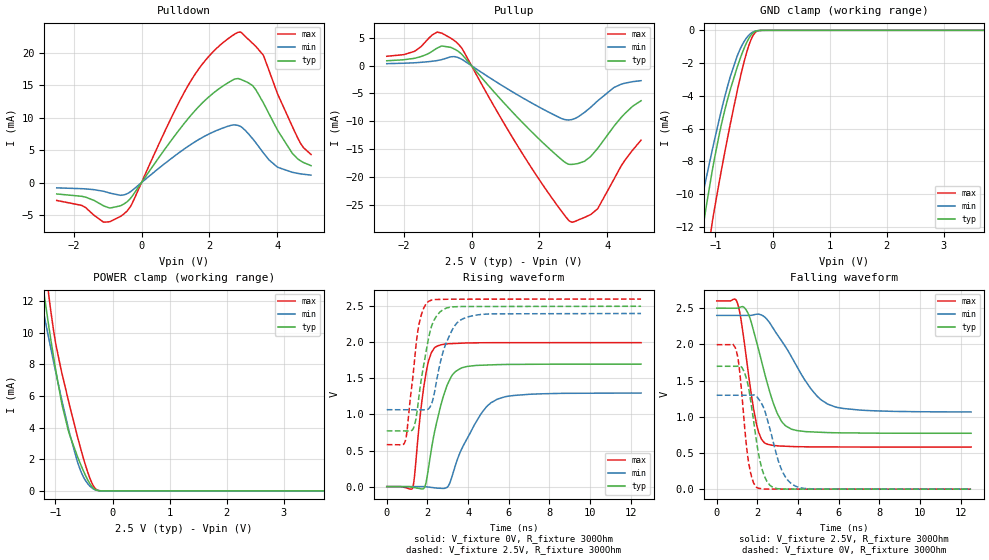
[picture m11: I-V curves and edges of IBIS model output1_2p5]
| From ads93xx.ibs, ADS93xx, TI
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|   output1_2p5 Model
[Model]   output1_2p5
Model_type   3-state
Polarity   Non-Inverting
Vmeas = 1.25
Vref = 0
Cref = 2pF
Rref = 100000
|   typ   min   max
C_comp   0.697pF   0.559pF   0.737pF
[Voltage Range]   2.5   2.4   2.6
[Temperature Range]   27   125   -40
[Pullup Reference]   2.5   2.4   2.6
[Pulldown Reference]   0   0   0
[Power Clamp Reference]   2.5   2.4   2.6
[GND Clamp Reference]   0   0   0
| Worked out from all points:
|   slope of the pulldown table from 0 to 0.375 V, typ, clamps not added: 132 ohm
|   slope of the pullup table from 0 to 0.375 V, typ, clamps not added: 139 ohm
|   GND clamp passes 1 mA (typ) near -0.49 V on its own axis
|   POWER clamp passes 1 mA (typ) near -0.48 V on its own axis
|   falling waveform, V_fixture 2.5V, R_fixture 300Ohm: 20-80 % time 1.03ns typ, 1.81ns min, 626ps max; typ from 2.5 V to 0.772 V
|   rising waveform, V_fixture 0V, R_fixture 300Ohm: 20-80 % time 812ps typ, 1.37ns min, 496ps max; typ from 0 V to 1.7 V
|   rising waveform, V_fixture 2.5V, R_fixture 300Ohm: 20-80 % time 609ps typ, 784ps min, 478ps max; typ from 0.772 V to 2.5 V
|   falling waveform, V_fixture 0V, R_fixture 300Ohm: 20-80 % time 578ps typ, 793ps min, 413ps max; typ from 1.7 V to 0 V
[Pulldown]
|   Voltage   I(typ)   I(min)   I(max)
-2.5V     -1.756mA   -815.4uA   -2.761mA
-1.758V   -2.121mA   -943.4uA   -3.53mA
-1.113V   -3.605mA   -1.354mA   -6.116mA
-512.5mV  -3.288mA   -1.893mA   -4.816mA
-280mV    -2.136mA   -1.231mA   -3.255mA
1.482V    10.54mA    5.976mA    15.93mA
2.112V    13.79mA    7.806mA    20.2mA
2.848V    16.06mA    8.824mA    23.21mA
3.275V    14.98mA    6.785mA    21.51mA
3.59V     12.34mA    4.612mA    19.68mA
4.445V    4.541mA    1.593mA    8.693mA
5V        2.616mA    1.152mA    4.337mA
[GND Clamp]
|   Voltage   I(typ)   I(min)   I(max)
-2.5V     -44.39mA   -33.12mA   -59.46mA
-1.413V   -16.56mA   -13.29mA   -21.57mA
-1.285V   -13.54mA   -11.09mA   -17.6mA
-1.21V    -11.83mA   -9.823mA   -15.46mA
-1.052V   -8.501mA   -7.252mA   -11.64mA
-865mV    -5.281mA   -4.442mA   -7.963mA
-737.5mV  -3.589mA   -2.797mA   -5.676mA
-617.5mV  -2.236mA   -1.555mA   -3.679mA
-452.5mV  -743.8uA   -449.7uA   -1.342mA
-332.5mV  -131.9uA   -85.99uA   -263.4uA
-197.5mV  -2.745uA   -3.997uA   -3.249uA
5V        0A         0A         0A
[Pullup]
|   Voltage   I(typ)   I(min)   I(max)
-2.5V     891.1uA    369.6uA    1.698mA
-1.705V   1.314mA    520.1uA    2.536mA
-1.015V   3.174mA    924.9uA    6.056mA
-407.5mV  2.663mA    1.498mA    4.016mA
1.587V    -10.76mA   -6.069mA   -16.67mA
2.652V    -16.89mA   -9.502mA   -26.19mA
2.953V    -17.78mA   -9.707mA   -28.18mA
3.335V    -17.21mA   -8.404mA   -27.33mA
3.717V    -14.92mA   -6.351mA   -25.78mA
4.205V    -10.87mA   -3.913mA   -20.4mA
4.527V    -8.597mA   -3.141mA   -17mA
5V        -6.311mA   -2.698mA   -13.41mA
[POWER Clamp]
|   Voltage   I(typ)   I(min)   I(max)
-2.5V     50.08mA    37.08mA    68.11mA
-1.292V   14.84mA    12.84mA    18.08mA
-1.248V   13.67mA    12.01mA    16.51mA
-1.202V   12.52mA    11.18mA    15mA
-1.113V   10.31mA    9.555mA    12.23mA
-992.5mV  7.585mA    7.466mA    9.256mA
-880mV    5.374mA    5.602mA    7.334mA
-775mV    3.82mA     3.973mA    5.74mA
-550mV    1.602mA    1.196mA    2.57mA
-407.5mV  524.1uA    345.2uA    909.1uA
-310mV    102.3uA    80.34uA    188.9uA
5V        0A         0A         0A
[Ramp]
R_load = 300
|   typ   min   max
dV/dt_r   1.01849/8.12329e-10   0.778351/1.37494e-09   1.19741/4.95737e-10
dV/dt_f   1.03672/1.03546e-09   0.800297/1.80824e-09   1.21089/6.25732e-10
[Falling Waveform]
V_fixture = 2.5V
V_fixture_min = 2.4V
V_fixture_max = 2.6V
R_fixture = 300Ohm
C_fixture = 0F
|   Time   V(typ)   V(min)   V(max)
0s        2.5V       2.4V       2.6V
1.014ns   2.5V       2.4V       2.572V
1.511ns   2.445V     2.4V       1.692V
1.942ns   2.05V      2.416V     917.2mV
2.389ns   1.561V     2.369V     632.5mV
2.962ns   1.055V     2.14V      599.4mV
3.382ns   874.9mV    1.965V     592.7mV
4.623ns   791.5mV    1.388V     584.2mV
5.449ns   781.5mV    1.176V     583.2mV
12.5ns    772.1mV    1.066V     581.8mV
[Rising Waveform]
V_fixture = 0V
V_fixture_min = 0V
V_fixture_max = 0V
R_fixture = 300Ohm
C_fixture = 0F
|   Time   V(typ)   V(min)   V(max)
0s        41.34nV    19.32uV    -152.7nV
1.273ns   -9.361mV   145.7uV    -18.99mV
1.679ns   -29.93mV   186uV      1.069V
1.942ns   72.44mV    -2.83mV    1.594V
2.485ns   926.3mV    -20.92mV   1.949V
3.008ns   1.43V      1.322mV    1.979V
3.382ns   1.597V     300.3mV    1.985V
4.623ns   1.682V     1.006V     1.994V
5.449ns   1.691V     1.214V     1.995V
12.5ns    1.697V     1.297V     1.996V
[Rising Waveform]
V_fixture = 2.5V
V_fixture_min = 2.4V
V_fixture_max = 2.6V
R_fixture = 300Ohm
C_fixture = 0F
|   Time   V(typ)   V(min)   V(max)
0s        772.1mV    1.066V     581.8mV
920.6ps   771.1mV    1.065V     640.5mV
1.322ns   815.1mV    1.065V     1.624V
1.542ns   1.157V     1.065V     2.182V
1.815ns   1.682V     1.065V     2.475V
2.059ns   2.062V     1.08V      2.569V
2.378ns   2.334V     1.353V     2.594V
2.902ns   2.471V     1.976V     2.597V
3.794ns   2.497V     2.333V     2.598V
12.5ns    2.5V       2.4V       2.6V
[Falling Waveform]
|Gnd
V_fixture = 0V
V_fixture_min = 0V
V_fixture_max = 0V
R_fixture = 300Ohm
C_fixture = 0F
|   Time   V(typ)   V(min)   V(max)
0s        1.697V     1.297V     1.996V
948.6ps   1.697V     1.297V     1.925V
1.098ns   1.702V     1.297V     1.698V
1.542ns   1.429V     1.297V     414.7mV
1.981ns   611.5mV    1.273V     21.41mV
2.245ns   259.6mV    1.161V     4.743mV
2.608ns   54.11mV    839.2mV    1.104mV
3.166ns   3.092mV    283.3mV    1.042mV
3.88ns    1.463mV    39.91mV    961.8uV
12.5ns    324.6nV    21.08uV    -203.9nV
